| IBIS file stm32mp211_213_215_vfbga361.ibs
[IBIS ver] 5.1
[File name] stm32mp211_213_215_vfbga361.ibs
[File Rev] 0.4
[Date] 09-10-2025
[Source] Data Created at STMicroelectronics
[Notes]  File originated from ELDO simulations.
[Disclaimer]  This information is for modeling purpose only and is
   not guaranted. The information is subject to change without
   notice.
[Copyright] Copyright 2025 STMicroelectronics Inc.
|   Component stm32mp211_213_215_vfbga361
[Component] stm32mp211_213_215_vfbga361
[Manufacturer] STMicroelectronics
[Package]
| variable   typ   min   max
R_pkg  0  NA  NA
L_pkg  0  NA  NA
C_pkg  0  NA  NA
[Pin]   signal_name   model_name
R5  ANA0  nc
P5  ANA1  nc
T2  BOOT0  isudq_tt
P3  BOOT1  isudq_tt
T3  BOOT2  isudq_tt
R3  BOOT3  isudq_tt
C2  CSI_CKN  DPHY_IBIS_L1
C1  CSI_CKP  DPHY_IBIS_L1
E1  CSI_D0N  DPHY_IBIS_L1
E2  CSI_D0P  DPHY_IBIS_L1
D2  CSI_D1N  DPHY_IBIS_L1
D1  CSI_D1P  DPHY_IBIS_L1
E3  CSI_REXT  nc
F17  DDR_A0  mal4drv20_PAD
G17  DDR_A1  mal4drv20_PAD
G18  DDR_A10  mal4drv20_PAD
F18  DDR_A11  mal4drv20_PAD
R17  DDR_A12  mal4drv20_PAD
J18  DDR_A13  mal4drv20_PAD
K18  DDR_A14  mal4drv20_PAD
L18  DDR_A15  mal4drv20_PAD
M18  DDR_A16  mal4drv20_PAD
N18  DDR_A17  mal4drv20_PAD
P18  DDR_A18  mal4drv20_PAD
J17  DDR_A2  mal4drv20_PAD
E19  DDR_A20  mal4drv20_PAD
F19  DDR_A21  mal4drv20_PAD
G19  DDR_A22  mal4drv20_PAD
H19  DDR_A23  mal4drv20_PAD
H17  DDR_A25  mal4drv20_PAD
K19  DDR_A26  mal4drv20_PAD
L19  DDR_A27  mal4drv20_PAD
M19  DDR_A28  mal4drv20_PAD
N19  DDR_A29  mal4drv20_PAD
J19  DDR_A3  mal4drv20_PAD
P19  DDR_A30  mal4drv20_PAD
R19  DDR_A31  mal4drv20_PAD
M17  DDR_A4  mal4drv20_PAD
L17  DDR_A5  mal4drv20_PAD
N17  DDR_A6  mal4drv20_PAD
P17  DDR_A7  mal4drv20_PAD
H18  DDR_A8  mal4drv20_PAD
E18  DDR_A9  mal4drv20_PAD
W18  DDR_DQ0  mal4drv27_PAD
W17  DDR_DQ1  mal4drv27_PAD
B17  DDR_DQ10  mal4drv27_PAD
A17  DDR_DQ11  mal4drv27_PAD
D19  DDR_DQ12  mal4drv27_PAD
D18  DDR_DQ13  mal4drv27_PAD
D17  DDR_DQ14  mal4drv27_PAD
C18  DDR_DQ15  mal4drv27_PAD
V17  DDR_DQ2  mal4drv27_PAD
U17  DDR_DQ3  mal4drv27_PAD
T19  DDR_DQ4  mal4drv27_PAD
T18  DDR_DQ5  mal4drv27_PAD
U19  DDR_DQ6  mal4drv27_PAD
U18  DDR_DQ7  mal4drv27_PAD
C17  DDR_DQ8  mal4drv27_PAD
A18  DDR_DQ9  mal4drv27_PAD
T17  DDR_DQM0  mal4drv27_PAD
C19  DDR_DQM1  mal4drv27_PAD
V18  DDR_DQS0N  mal4drv27_PAD
V19  DDR_DQS0P  mal4drv27_PAD
B18  DDR_DQS1N  mal4drv27_PAD
B19  DDR_DQS1P  mal4drv27_PAD
E17  DDR_RESETN  nc
K17  DDR_VREF  nc
G16  DDR_ZQ  nc
W4  JTCK_SWCLK  io8_tt
W3  JTDI  io8_tt
V1  JTDO_TRACESWO  io8_tt
W2  JTMS_SWDIO  io8_tt
V2  NJTRST  io8_tt
N2  NRST  nc
T1  NRSTC1MS  io8_tt
R1  OSC_IN  isudq_v18
R2  OSC_OUT  isudq_v18
M2  OSC32_IN  isudq_v18
M1  OSC32_OUT  isudq_v18
V12  OTG_HSDM  USB2_HS_IBIS
W12  OTG_HSDP  USB2_HS_IBIS
R15  OTG_TXRTUNE  nc
P15  PA0  io8_tt
N15  PA1  io8_tt_i3c
M15  PA10  io8_tt
R9  PA11  io8_tt
R8  PA12  io8_tt_i3c
W9  PA13  io8_tt
T8  PA14  io8_tt
T10  PA15  io8_tt_i3c
N12  PA2  io8_tt_i3c
R12  PA3  io8_tt_i3c
P12  PA4  io8_tt
J12  PA5  io8_tt
M14  PA6  io8_tt
K15  PA7  io8_tt
K9  PA8  io8_tt_i3c
K12  PA9  io8_tt
D9  PB1  io8_tt
E12  PB10  io8_tt
B7  PB11  io8_tt
E14  PB12  io8_tt
G15  PB13  io8_tt
H15  PB14  io8_tt
J15  PB15  io8_tt
E9  PB2  io8_tt
A9  PB3  io8_tt
B9  PB5  io8_tt_i3c
C8  PB6  io8_tt
D7  PB7  io8_tt
A8  PB9  io8_tt
V9  PC0  io8_tt
V10  PC1  io8_tt_i3c
W6  PC10  io8_tt
V5  PC11  io8_tt
V4  PC12  io8_tt_i3c
P4  PC13  io8_tt
T9  PC2  io8_tt
U4  PC3  io8_tt
V3  PC4  io8_tt
T7  PC5  io8_tt_i3c
R7  PC6  io8_tt_i3c
W5  PC7  io8_tt
U6  PC8  io8_tt
V6  PC9  io8_tt
C11  PD0  io8_tt
F9  PD1  io8_tt
D11  PD10  io8_tt_i3c
B10  PD11  io8_tt_i3c
H14  PD12  io8_tt
G9  PD13  io8_tt
A13  PD14  io8_tt
A11  PD15  io8_tt_i3c
A10  PD2  io8_tt
D8  PD3  io8_tt
C12  PD4  io8_tt
B12  PD5  io8_tt
A12  PD6  io8_tt
D12  PD7  io8_tt
E11  PD8  io8_tt
C10  PD9  io8_tt
N1  PDR_ON  nc
B13  PE0  io8_tt
C13  PE1  io8_tt
D15  PE10  io8_tt
B16  PE11  io8_tt
C16  PE12  io8_tt
A16  PE13  io8_tt
G14  PE14  io8_tt
D14  PE15  io8_tt
A14  PE2  io8_tt
A15  PE3  io8_tt
B14  PE4  io8_tt
C14  PE5  io8_tt
F14  PE6  io8_tt
C15  PE7  io8_tt
B15  PE8  io8_tt
F15  PE9  io8_tt
N9  PF0  io8_tt_i3c
U8  PF1  io8_tt
L9  PF10  io8_tt
T4  PF11  io8_tt
L7  PF12  io8_tt
H2  PF13  io8_tt
G5  PF15  io8_tt
P9  PF2  io8_tt_i3c
W10  PF3  io8_tt
W7  PF4  io8_tt
P7  PF5  io8_tt
U5  PF6  io8_tt
V7  PF7  io8_tt
U7  PF8  io8_tt
T6  PF9  io8_tt
T5  PG0  io8_tt_i3c
R4  PG1  io8_tt_i3c
F5  PG10  io8_tt
F7  PG11  io8_tt
H7  PG12  io8_tt
J7  PG13  io8_tt_i3c
H5  PG14  io8_tt
E4  PG15  io8_tt
M7  PG2  io8_tt_i3c
H12  PG3  io8_tt
N7  PG4  io8_tt
K1  PG5  io8_tt
E7  PG7  io8_tt
E5  PG8  io8_tt
G2  PG9  io8_tt
U10  PH10  io8_tt
T11  PH11  io8_tt
V8  PH12  io8_tt
U9  PH13  io8_tt
G12  PH4  io8_tt
M9  PH5  io8_tt
L12  PH7  io8_tt
M12  PH8  io8_tt
W8  PH9  io8_tt
H1  PI0  io8_tt
J9  PI1  io8_tt_i3c
G1  PI4  io8_tt
K7  PI5  io8_tt
D4  PI6  io8_tt
N4  PI8  io8_tt
P2  PWR_CPUON  io8_tt
P1  PWR_LP  io8_tt
U3  PWR_ON  io8_tt
L5  PZ0  io8_tt_i3c_tamp
M4  PZ1  io8_tt_i3c_tamp
M5  PZ3  io8_tt_i3c_tamp
V11  USBH_HS_DM  USB2_HS_IBIS
W11  USBH_HS_DP  USB2_HS_IBIS
T15  USBH_HS_TXRTUNE  nc
M8  V08CAP  nc
R6  VBAT  power
H8  VDD  power
K8  VDD  power
L6  VDD  power
R14  VDD33USB  power
N6  VDDA18ADC  power
N5  VDDA18AON  power
D3  VDDA18CSI  power
D16  VDDA18DDR  nc
E15  VDDA18PLL1  nc
G6  VDDA18PLL2  nc
T13  VDDA18USB  power
G10  VDDCORE  nc
H11  VDDCORE  nc
J10  VDDCORE  nc
K11  VDDCORE  nc
L10  VDDCORE  nc
M11  VDDCORE  nc
N8  VDDCORE  nc
N10  VDDCORE  nc
N14  VDDCORE  nc
P11  VDDCORE  nc
P13  VDDCORE  nc
R10  VDDCORE  nc
E13  VDDCPU  nc
G13  VDDCPU  nc
J13  VDDCPU  nc
L13  VDDCPU  nc
M13  VDDCPU  nc
B1  VDDCSI  nc
D10  VDDIO1  power
F8  VDDIO2  power
E10  VDDIO3  power
F10  VDDIO3  power
F16  VDDQDDR  power
J16  VDDQDDR  power
L16  VDDQDDR  power
M16  VDDQDDR  power
P16  VDDQDDR  power
T16  VDDQDDR  power
U1  VREFN  nc
U2  VREFP  nc
A1  VSS  gnd
A19  VSS  gnd
C3  VSS  gnd
C7  VSS  gnd
D13  VSS  gnd
E8  VSS  gnd
E16  VSS  gnd
F6  VSS  gnd
F11  VSS  gnd
F13  VSS  gnd
G8  VSS  gnd
G11  VSS  gnd
H10  VSS  gnd
H13  VSS  gnd
H16  VSS  gnd
J6  VSS  gnd
J8  VSS  gnd
J11  VSS  gnd
J14  VSS  gnd
K4  VSS  gnd
K5  VSS  gnd
K10  VSS  gnd
K13  VSS  gnd
K16  VSS  gnd
L8  VSS  gnd
L11  VSS  gnd
M10  VSS  gnd
N11  VSS  gnd
N13  VSS  gnd
N16  VSS  gnd
P8  VSS  gnd
P10  VSS  gnd
P14  VSS  gnd
R11  VSS  gnd
R16  VSS  gnd
R18  VSS  gnd
W1  VSS  gnd
W19  VSS  gnd
P6  VSSA  nc
M6  VSSAON  nc
[Package Model]   503-fcvfbga-10x10-361-240814
[Pin Mapping]   pulldown_ref   pullup_ref   | Comment
R5  nc  nc
P5  nc  nc
T2  gnd  vdd
P3  gnd  vdd
T3  gnd  vdd
R3  gnd  vdd
C2  gnd  VDDA18CSI
C1  gnd  VDDA18CSI
E1  gnd  VDDA18CSI
E2  gnd  VDDA18CSI
D2  gnd  VDDA18CSI
D1  gnd  VDDA18CSI
E3  nc  nc
F17  gnd  vddqddr
G17  gnd  vddqddr
G18  gnd  vddqddr
F18  gnd  vddqddr
R17  gnd  vddqddr
J18  gnd  vddqddr
K18  gnd  vddqddr
L18  gnd  vddqddr
M18  gnd  vddqddr
N18  gnd  vddqddr
P18  gnd  vddqddr
J17  gnd  vddqddr
E19  gnd  vddqddr
F19  gnd  vddqddr
G19  gnd  vddqddr
H19  gnd  vddqddr
H17  gnd  vddqddr
K19  gnd  vddqddr
L19  gnd  vddqddr
M19  gnd  vddqddr
N19  gnd  vddqddr
J19  gnd  vddqddr
P19  gnd  vddqddr
R19  gnd  vddqddr
M17  gnd  vddqddr
L17  gnd  vddqddr
N17  gnd  vddqddr
P17  gnd  vddqddr
H18  gnd  vddqddr
E18  gnd  vddqddr
W18  gnd  vddqddr
W17  gnd  vddqddr
B17  gnd  vddqddr
A17  gnd  vddqddr
D19  gnd  vddqddr
D18  gnd  vddqddr
D17  gnd  vddqddr
C18  gnd  vddqddr
V17  gnd  vddqddr
U17  gnd  vddqddr
T19  gnd  vddqddr
T18  gnd  vddqddr
U19  gnd  vddqddr
U18  gnd  vddqddr
C17  gnd  vddqddr
A18  gnd  vddqddr
T17  gnd  vddqddr
C19  gnd  vddqddr
V18  gnd  vddqddr
V19  gnd  vddqddr
B18  gnd  vddqddr
B19  gnd  vddqddr
E17  nc  nc
K17  nc  nc
G16  nc  nc
W4  gnd  vdd
W3  gnd  vdd
V1  gnd  vdd
W2  gnd  vdd
V2  gnd  vdd
N2  nc  nc
T1  gnd  vdd
R1  gnd  vdda18aon
R2  gnd  vdda18aon
M2  gnd  vdd  | Depending on IO usage
| M2  gnd  vsw  | Depending on IO usage
M1  gnd  vdd  | Depending on IO usage
| M1  gnd  vsw  | Depending on IO usage
V12  gnd  VDD33USB
W12  gnd  VDD33USB
R15  nc  nc
P15  gnd  vdd
N15  gnd  vdd
M15  gnd  vdd
R9  gnd  vdd
R8  gnd  vdd
W9  gnd  vdd
T8  gnd  vdd
T10  gnd  vdd
N12  gnd  vdd
R12  gnd  vdd
P12  gnd  vdd
J12  gnd  vdd
M14  gnd  vdd
K15  gnd  vdd
K9  gnd  vdd
K12  gnd  vdd
D9  gnd  vdd
E12  gnd  vdd
B7  gnd  vdd
E14  gnd  vdd
G15  gnd  vdd
H15  gnd  vdd
J15  gnd  vdd
E9  gnd  vdd
A9  gnd  vdd
B9  gnd  vdd
C8  gnd  vdd
D7  gnd  vdd
A8  gnd  vdd
V9  gnd  vdd
V10  gnd  vdd
W6  gnd  vdd
V5  gnd  vdd
V4  gnd  vdd
P4  gnd  vdd  | Depending on IO usage
| P4  gnd  vsw  | Depending on IO usage
T9  gnd  vdd
U4  gnd  vdd
V3  gnd  vdd
T7  gnd  vdd
R7  gnd  vdd
W5  gnd  vdd
U6  gnd  vdd
V6  gnd  vdd
C11  gnd  vddio3
F9  gnd  vddio3
D11  gnd  vddio3
B10  gnd  vddio3
H14  gnd  vdd
G9  gnd  vdd
A13  gnd  vdd
A11  gnd  vdd
A10  gnd  vddio3
D8  gnd  vddio3
C12  gnd  vddio3
B12  gnd  vddio3
A12  gnd  vddio3
D12  gnd  vddio3
E11  gnd  vddio3
C10  gnd  vddio3
N1  nc  nc
B13  gnd  vddio1
C13  gnd  vddio1
D15  gnd  vddio2
B16  gnd  vddio2
C16  gnd  vddio2
A16  gnd  vddio2
G14  gnd  vddio2
D14  gnd  vddio2
A14  gnd  vddio1
A15  gnd  vddio1
B14  gnd  vddio1
C14  gnd  vddio1
F14  gnd  vddio1
C15  gnd  vddio1
B15  gnd  vddio1
F15  gnd  vddio1
N9  gnd  vdd
U8  gnd  vdd
L9  gnd  vdd
T4  gnd  vdd
L7  gnd  vdd
H2  gnd  vdd
G5  gnd  vdd
P9  gnd  vdd
W10  gnd  vdd
W7  gnd  vdd
P7  gnd  vdd
U5  gnd  vdd
V7  gnd  vdd
U7  gnd  vdd
T6  gnd  vdd
T5  gnd  vdd
R4  gnd  vdd
F5  gnd  vdd
F7  gnd  vdd
H7  gnd  vdd
J7  gnd  vdd
H5  gnd  vdd
E4  gnd  vdd
M7  gnd  vdd
H12  gnd  vdd
N7  gnd  vdd
K1  gnd  vdd
E7  gnd  vdd
E5  gnd  vdd
G2  gnd  vdd
U10  gnd  vdd
T11  gnd  vdd
V8  gnd  vdd
U9  gnd  vdd
G12  gnd  vdd
M9  gnd  vdd
L12  gnd  vdd
M12  gnd  vdd
W8  gnd  vdd
H1  gnd  vdd
J9  gnd  vdd
G1  gnd  vdd
K7  gnd  vdd
D4  gnd  vdd
N4  gnd  vdd
P2  gnd  vdd
P1  gnd  vdd
U3  gnd  vdd
L5  gnd  vdd  | Depending on IO usage
| L5  gnd  vsw  | Depending on IO usage
M4  gnd  vdd  | Depending on IO usage
| M4  gnd  vsw  | Depending on IO usage
M5  gnd  vdd  | Depending on IO usage
| M5  gnd  vsw  | Depending on IO usage
V11  gnd  VDD33USB
W11  gnd  VDD33USB
T15  nc  nc
M8  nc  nc
R6  nc  vsw
H8  nc  vdd
K8  nc  vdd
L6  nc  vdd
R14  nc  VDD33USB
N6  nc  vdda18adc
N5  nc  vdda18aon
D3  nc  VDDA18CSI
D16  nc  nc
E15  nc  nc
G6  nc  nc
T13  nc  vdda18usb
G10  nc  nc
H11  nc  nc
J10  nc  nc
K11  nc  nc
L10  nc  nc
M11  nc  nc
N8  nc  nc
N10  nc  nc
N14  nc  nc
P11  nc  nc
P13  nc  nc
R10  nc  nc
E13  nc  nc
G13  nc  nc
J13  nc  nc
L13  nc  nc
M13  nc  nc
B1  nc  nc
D10  nc  vddio1
F8  nc  vddio2
E10  nc  vddio3
F10  nc  vddio3
F16  nc  vddqddr
J16  nc  vddqddr
L16  nc  vddqddr
M16  nc  vddqddr
P16  nc  vddqddr
T16  nc  vddqddr
U1  nc  nc
U2  nc  nc
A1  gnd  nc
A19  gnd  nc
C3  gnd  nc
C7  gnd  nc
D13  gnd  nc
E8  gnd  nc
E16  gnd  nc
F6  gnd  nc
F11  gnd  nc
F13  gnd  nc
G8  gnd  nc
G11  gnd  nc
H10  gnd  nc
H13  gnd  nc
H16  gnd  nc
J6  gnd  nc
J8  gnd  nc
J11  gnd  nc
J14  gnd  nc
K4  gnd  nc
K5  gnd  nc
K10  gnd  nc
K13  gnd  nc
K16  gnd  nc
L8  gnd  nc
L11  gnd  nc
M10  gnd  nc
N11  gnd  nc
N13  gnd  nc
N16  gnd  nc
P8  gnd  nc
P10  gnd  nc
P14  gnd  nc
R11  gnd  nc
R16  gnd  nc
R18  gnd  nc
W1  gnd  nc
W19  gnd  nc
P6  nc  nc
M6  nc  nc
[Diff Pin]  inv_pin  vdiff  tdelay_typ  tdelay_min  tdelay_max
C2  C1  NA  NA  NA  NA
E1  E2  NA  NA  NA  NA
D2  D1  NA  NA  NA  NA
V19  V18  NA  NA  NA  NA
B19  B18  NA  NA  NA  NA
W11  V11  NA  NA  NA  NA   |USBH_HS_DP _DM
W12  V12  NA  NA  NA  NA   |USBH_HS_DP _DM
M17  L17  NA  NA  NA  NA
[Model Selector] USB2_HS_IBIS
USB2_HSRX   USB2 HSRX model
USB2_HSTX_00_0_01_0011_11   TuningBits_AMP_PULSE_RISE_REF_XV=00_0_01_0011_11
USB2_HSTX_00_0_10_0101_11   TuningBits_AMP_PULSE_RISE_REF_XV=00_0_10_0101_11
USB2_HSTX_00_0_11_0111_11   TuningBits_AMP_PULSE_RISE_REF_XV=00_0_11_0111_11
USB2_HSTX_00_1_01_0011_11   TuningBits_AMP_PULSE_RISE_REF_XV=00_1_01_0011_11
USB2_HSTX_00_1_10_0101_11   TuningBits_AMP_PULSE_RISE_REF_XV=00_1_10_0101_11
USB2_HSTX_00_1_11_0111_11   TuningBits_AMP_PULSE_RISE_REF_XV=00_1_11_0111_11
USB2_HSTX_01_0_01_0011_11   TuningBits_AMP_PULSE_RISE_REF_XV=01_0_01_0011_11
USB2_HSTX_01_0_10_0101_11   TuningBits_AMP_PULSE_RISE_REF_XV=01_0_10_0101_11
USB2_HSTX_01_0_11_0111_11   TuningBits_AMP_PULSE_RISE_REF_XV=01_0_11_0111_11
USB2_HSTX_01_1_01_0011_11   TuningBits_AMP_PULSE_RISE_REF_XV=01_1_01_0011_11
USB2_HSTX_01_1_10_0101_11   TuningBits_AMP_PULSE_RISE_REF_XV=01_1_10_0101_11
USB2_HSTX_01_1_11_0111_11   TuningBits_AMP_PULSE_RISE_REF_XV=01_1_11_0111_11
USB2_HSTX_10_0_01_0011_11   TuningBits_AMP_PULSE_RISE_REF_XV=10_0_01_0011_11
USB2_HSTX_10_0_10_0101_11   TuningBits_AMP_PULSE_RISE_REF_XV=10_0_10_0101_11
USB2_HSTX_10_0_11_0111_11   TuningBits_AMP_PULSE_RISE_REF_XV=10_0_11_0111_11
USB2_HSTX_10_1_01_0011_11   TuningBits_AMP_PULSE_RISE_REF_XV=10_1_01_0011_11
USB2_HSTX_10_1_10_0101_11   TuningBits_AMP_PULSE_RISE_REF_XV=10_1_10_0101_11
USB2_HSTX_10_1_11_0111_11   TuningBits_AMP_PULSE_RISE_REF_XV=10_1_11_0111_11
[Model Selector] DPHY_IBIS_L1
DPHY_RX_2P5G_L1   DPHY HSRX model at 2.5Gbps for lane 1
DPHY_RX_1P5G_L1   DPHY HSRX model at 1.5Gbps for lane 1
[Model Selector] io8_tt
io8_tt_ls_3v3 "GPIO - 3V tolerant - low speed - 3.3V range"
io8_tt_ms_3v3 "GPIO - 3V tolerant - med speed - 3.3V range"
io8_tt_fs_3v3 "GPIO - 3V tolerant - fast speed - 3.3V range"
io8_tt_hs_3v3 "GPIO - 3V tolerant - high speed - 3.3V range"
io8_tt_hslv_ls_1v8 "GPIO low voltage optimization - 3V tolerant - low speed - 1.8V range"
io8_tt_hslv_ms_1v8 "GPIO low voltage optimization - 3V tolerant - med speed - 1.8V range"
io8_tt_hslv_fs_1v8 "GPIO low voltage optimization - 3V tolerant - fast speed - 1.8V range"
io8_tt_hslv_hs_1v8 "GPIO low voltage optimization - 3V tolerant - high speed - 1.8V range"
[Model Selector] io8_tt_i3c
io8_tt_ls_3v3 "GPIO - 3V tolerant - low speed - 3.3V range"
io8_tt_ms_3v3 "GPIO - 3V tolerant - med speed - 3.3V range"
io8_tt_fs_3v3 "GPIO - 3V tolerant - fast speed - 3.3V range"
io8_tt_hs_3v3 "GPIO - 3V tolerant - high speed - 3.3V range"
io8_tt_hslv_ls_1v8 "GPIO low voltage optimization - 3V tolerant - low speed - 1.8V range"
io8_tt_hslv_ms_1v8 "GPIO low voltage optimization - 3V tolerant - med speed - 1.8V range"
io8_tt_hslv_fs_1v8 "GPIO low voltage optimization - 3V tolerant - fast speed - 1.8V range"
io8_tt_hslv_hs_1v8 "GPIO low voltage optimization - 3V tolerant - high speed - 1.8V range"
io8_tt_i3c_ls_3v3 "GPIO with I3C open-drain - 3V tolerant - low speed - 3.3V range"
io8_tt_i3c_ms_3v3 "GPIO with I3C open-drain - 3V tolerant - med speed - 3.3V range"
io8_tt_i3c_fs_3v3 "GPIO with I3C open-drain - 3V tolerant - fast speed - 3.3V range"
io8_tt_i3c_hs_3v3 "GPIO with I3C open-drain - 3V tolerant - high speed - 3.3V range"
io8_tt_hslv_i3c_ls_1v8 "GPIO low voltage optimization with I3C open-drain - 3V tolerant - low speed - 1.8V range"
io8_tt_hslv_i3c_ms_1v8 "GPIO low voltage optimization with I3C open-drain - 3V tolerant - med speed - 1.8V range"
io8_tt_hslv_i3c_fs_1v8 "GPIO low voltage optimization with I3C open-drain - 3V tolerant - fast speed - 1.8V range"
io8_tt_hslv_i3c_hs_1v8 "GPIO low voltage optimization with I3C open-drain - 3V tolerant - high speed - 1.8V range"
io8_tt_i3c_fmp_3v3 "GPIO with I3C fm+ open-drain - 3V tolerant - 3.3V range"
[Model Selector] io8_tt_i3c_tamp
io8_tt_ls_3v3 "GPIO - 3V tolerant - low speed - 3.3V range"
io8_tt_ms_3v3 "GPIO - 3V tolerant - med speed - 3.3V range"
io8_tt_fs_3v3 "GPIO - 3V tolerant - fast speed - 3.3V range"
io8_tt_hs_3v3 "GPIO - 3V tolerant - high speed - 3.3V range"
io8_tt_hslv_ls_1v8 "GPIO low voltage optimization - 3V tolerant - low speed - 1.8V range"
io8_tt_hslv_ms_1v8 "GPIO low voltage optimization - 3V tolerant - med speed - 1.8V range"
io8_tt_hslv_fs_1v8 "GPIO low voltage optimization - 3V tolerant - fast speed - 1.8V range"
io8_tt_hslv_hs_1v8 "GPIO low voltage optimization - 3V tolerant - high speed - 1.8V range"
io8_tt_i3c_ls_3v3 "GPIO with I3C open-drain - 3V tolerant - low speed - 3.3V range"
io8_tt_i3c_ms_3v3 "GPIO with I3C open-drain - 3V tolerant - med speed - 3.3V range"
io8_tt_i3c_fs_3v3 "GPIO with I3C open-drain - 3V tolerant - fast speed - 3.3V range"
io8_tt_i3c_hs_3v3 "GPIO with I3C open-drain - 3V tolerant - high speed - 3.3V range"
io8_tt_hslv_i3c_ls_1v8 "GPIO low voltage optimization with I3C open-drain - 3V tolerant - low speed - 1.8V range"
io8_tt_hslv_i3c_ms_1v8 "GPIO low voltage optimization with I3C open-drain - 3V tolerant - med speed - 1.8V range"
io8_tt_hslv_i3c_fs_1v8 "GPIO low voltage optimization with I3C open-drain - 3V tolerant - fast speed - 1.8V range"
io8_tt_hslv_i3c_hs_1v8 "GPIO low voltage optimization with I3C open-drain - 3V tolerant - high speed - 1.8V range"
io8_tt_i3c_fmp_3v3 "GPIO with I3C fm+ open-drain - 3V tolerant - 3.3V range"
io8_tt_tamp_3v3 "IO tamper - 3V tolerant - 3.3V range"
io8_tt_tamp_1v8 "IO tamper - 3V tolerant - 1.8V range"
[Model Selector] isudq_tt
isudq_tt_3v3 "Input Buffer - 3V tolerant - 3.3V range"
isudq_tt_1v8 "Input Buffer - 3V tolerant - 1.8V range"
|[Model Selector] isudq_v18
|isudq_v18_1v8 "Input Buffer - 1.8V range "
[Model Selector]   mal4drv20_PAD
mal4drv20_d3l_40   DDR3L mal4drv20 cell  Z0=40-Ohm Driver
mal4drv20_d3l_60   DDR3L mal4drv20 cell  Z0=60-Ohm Driver
mal4drv20_d3l_120   DDR3L mal4drv20 cell  Z0=120-Ohm Driver
mal4drv20_d3_20   DDR3 mal4drv20 cell  Z0=20-Ohm Driver
mal4drv20_d3_24   DDR3 mal4drv20 cell  Z0=24-Ohm Driver
mal4drv20_d3_30   DDR3 mal4drv20 cell  Z0=30-Ohm Driver
mal4drv20_d3_40   DDR3 mal4drv20 cell  Z0=40-Ohm Driver
mal4drv20_d3_60   DDR3 mal4drv20 cell  Z0=60-Ohm Driver
mal4drv20_d4_20   DDR4 mal4drv20 cell  Z0=20-Ohm Driver
mal4drv20_d4_24   DDR4 mal4drv20 cell  Z0=24-Ohm Driver
mal4drv20_d4_30   DDR4 mal4drv20 cell  Z0=30-Ohm Driver
mal4drv20_d4_40   DDR4 mal4drv20 cell  Z0=40-Ohm Driver
mal4drv20_d4_60   DDR4 mal4drv20 cell  Z0=60-Ohm Driver
mal4drv20_dl4_20   LPDDR4 mal4drv20 cell  Z0=20-Ohm Driver
mal4drv20_dl4_24   LPDDR4 mal4drv20 cell  Z0=24-Ohm Driver
mal4drv20_dl4_30   LPDDR4 mal4drv20 cell  Z0=30-Ohm Driver
mal4drv20_dl4_40   LPDDR4 mal4drv20 cell  Z0=40-Ohm Driver
mal4drv20_dl4_60   LPDDR4 mal4drv20 cell  Z0=60-Ohm Driver
[Model Selector]   mal4drv27_PAD
mal4drv27_d3l_40   DDR3L mal4drv27 cell  Z0=40-Ohm Driver
mal4drv27_d3l_48   DDR3L mal4drv27 cell  Z0=48-Ohm Driver
mal4drv27_d3l_60   DDR3L mal4drv27 cell  Z0=60-Ohm Driver
mal4drv27_d3l_80   DDR3L mal4drv27 cell  Z0=80-Ohm Driver
mal4drv27_d3l_120   DDR3L mal4drv27 cell  Z0=120-Ohm Driver
mal4drv27_d3l_240   DDR3L mal4drv27 cell  Z0=240-Ohm Driver
mal4drv27_d3l_odt120   DDR3L mal4drv27 cell 120-Ohm ODT Receiver
mal4drv27_d3l_odt60   DDR3L mal4drv27 cell 60-Ohm ODT Receiver
mal4drv27_d3l_odtoff   DDR3L mal4drv27 cell ODT OFF Receiver
mal4drv27_d3_28   DDR3 mal4drv27 cell  Z0=28-Ohm Driver
mal4drv27_d3_34   DDR3 mal4drv27 cell  Z0=34-Ohm Driver
mal4drv27_d3_40   DDR3 mal4drv27 cell  Z0=40-Ohm Driver
mal4drv27_d3_53   DDR3 mal4drv27 cell  Z0=53-Ohm Driver
mal4drv27_d3_odt120   DDR3 mal4drv27 cell 120-Ohm ODT Receiver
mal4drv27_d3_odt60   DDR3 mal4drv27 cell 60-Ohm ODT Receiver
mal4drv27_d4_28   DDR4 mal4drv27 cell  Z0=28-Ohm Driver
mal4drv27_d4_34   DDR4 mal4drv27 cell  Z0=34-Ohm Driver
mal4drv27_d4_40   DDR4 mal4drv27 cell  Z0=40-Ohm Driver
mal4drv27_d4_53   DDR4 mal4drv27 cell  Z0=53-Ohm Driver
mal4drv27_d4_odt120   DDR4 mal4drv27 cell 120-Ohm ODT Receiver
mal4drv27_d4_odt240   DDR4 mal4drv27 cell 240-Ohm ODT Receiver
mal4drv27_d4_odt48   DDR4 mal4drv27 cell 48-Ohm ODT Receiver
mal4drv27_d4_odt60   DDR4 mal4drv27 cell 60-Ohm ODT Receiver
mal4drv27_d4_odt80   DDR4 mal4drv27 cell 80-Ohm ODT Receiver
mal4drv27_dl4_28   LPDDR4 mal4drv27 cell  Z0=28-Ohm Driver
mal4drv27_dl4_34   LPDDR4 mal4drv27 cell  Z0=34-Ohm Driver
mal4drv27_dl4_40   LPDDR4 mal4drv27 cell  Z0=40-Ohm Driver
mal4drv27_dl4_53   LPDDR4 mal4drv27 cell  Z0=53-Ohm Driver
mal4drv27_dl4_odt48   LPDDR4 mal4drv27 cell 48-Ohm ODT Receiver
mal4drv27_dl4_odt60   LPDDR4 mal4drv27 cell 60-Ohm ODT Receiver
[Define Package Model]  503-fcvfbga-10x10-361-240814
[Manufacturer]  unknown
[OEM]  unknown
[Description]  unknown
[Number Of Pins]  235
[Pin Numbers]
| Pin Name Terminal   Net Name   Starting Node   Ending Node
R5 | ANA0
P5 | ANA1
T2 | BOOT0
P3 | BOOT1
T3 | BOOT2
R3 | BOOT3
C2 | CSI_CKN
C1 | CSI_CKP
E1 | CSI_D0N
E2 | CSI_D0P
D2 | CSI_D1N
D1 | CSI_D1P
E3 | CSI_REXT
F17 | DDR_A0
G17 | DDR_A1
J17 | DDR_A2
J19 | DDR_A3
M17 | DDR_A4
L17 | DDR_A5
N17 | DDR_A6
P17 | DDR_A7
H18 | DDR_A8
E18 | DDR_A9
G18 | DDR_A10
F18 | DDR_A11
R17 | DDR_A12
J18 | DDR_A13
K18 | DDR_A14
L18 | DDR_A15
M18 | DDR_A16
N18 | DDR_A17
P18 | DDR_A18
E19 | DDR_A20
F19 | DDR_A21
G19 | DDR_A22
H19 | DDR_A23
H17 | DDR_A25
K19 | DDR_A26
L19 | DDR_A27
M19 | DDR_A28
N19 | DDR_A29
P19 | DDR_A30
R19 | DDR_A31
W18 | DDR_DQ0
W17 | DDR_DQ1
V17 | DDR_DQ2
U17 | DDR_DQ3
T19 | DDR_DQ4
T18 | DDR_DQ5
U19 | DDR_DQ6
U18 | DDR_DQ7
C17 | DDR_DQ8
A18 | DDR_DQ9
B17 | DDR_DQ10
A17 | DDR_DQ11
D19 | DDR_DQ12
D18 | DDR_DQ13
D17 | DDR_DQ14
C18 | DDR_DQ15
T17 | DDR_DQM0
C19 | DDR_DQM1
V18 | DDR_DQS0N
V19 | DDR_DQS0P
B18 | DDR_DQS1N
B19 | DDR_DQS1P
E17 | DDR_RESETN
K17 | DDR_VREF
G16 | DDR_ZQ
W4 | JTCK_SWCLK
W3 | JTDI
V1 | JTDO_TRACESWO
W2 | JTMS_SWDIO
V2 | NJTRST
N2 | NRST
T1 | NRSTC1MS
M2 | OSC32_IN
M1 | OSC32_OUT
R1 | OSC_IN
R2 | OSC_OUT
V12 | OTG_HSDM
W12 | OTG_HSDP
R15 | OTG_TXRTUNE
P15 | PA0
N15 | PA1
N12 | PA2
R12 | PA3
P12 | PA4
J12 | PA5
M14 | PA6
K15 | PA7
K9 | PA8
K12 | PA9
M15 | PA10
R9 | PA11
R8 | PA12
W9 | PA13
T8 | PA14
T10 | PA15
D9 | PB1
E9 | PB2
A9 | PB3
B9 | PB5
C8 | PB6
D7 | PB7
A8 | PB9
E12 | PB10
B7 | PB11
E14 | PB12
G15 | PB13
H15 | PB14
J15 | PB15
V9 | PC0
V10 | PC1
T9 | PC2
U4 | PC3
V3 | PC4
T7 | PC5
R7 | PC6
W5 | PC7
U6 | PC8
V6 | PC9
W6 | PC10
V5 | PC11
V4 | PC12
P4 | PC13
C11 | PD0
F9 | PD1
A10 | PD2
D8 | PD3
C12 | PD4
B12 | PD5
A12 | PD6
D12 | PD7
E11 | PD8
C10 | PD9
D11 | PD10
B10 | PD11
H14 | PD12
G9 | PD13
A13 | PD14
A11 | PD15
N1 | PDR_ON
B13 | PE0
C13 | PE1
A14 | PE2
A15 | PE3
B14 | PE4
C14 | PE5
F14 | PE6
C15 | PE7
B15 | PE8
F15 | PE9
D15 | PE10
B16 | PE11
C16 | PE12
A16 | PE13
G14 | PE14
D14 | PE15
N9 | PF0
U8 | PF1
P9 | PF2
W10 | PF3
W7 | PF4
P7 | PF5
U5 | PF6
V7 | PF7
U7 | PF8
T6 | PF9
L9 | PF10
T4 | PF11
L7 | PF12
H2 | PF13
G5 | PF15
T5 | PG0
R4 | PG1
M7 | PG2
H12 | PG3
N7 | PG4
K1 | PG5
E7 | PG7
E5 | PG8
G2 | PG9
F5 | PG10
F7 | PG11
H7 | PG12
J7 | PG13
H5 | PG14
E4 | PG15
G12 | PH4
M9 | PH5
L12 | PH7
M12 | PH8
W8 | PH9
U10 | PH10
T11 | PH11
V8 | PH12
U9 | PH13
H1 | PI0
J9 | PI1
G1 | PI4
K7 | PI5
D4 | PI6
N4 | PI8
P2 | PWR_CPUON
P1 | PWR_LP
U3 | PWR_ON
L5 | PZ0
M4 | PZ1
M5 | PZ3
V11 | USBH_HS_DM
W11 | USBH_HS_DP
T15 | USBH_HS_TXRTUNE
M8 | V08CAP
R6 | VBAT
R14 | VDD33USB
H8 | VDD
N6 | VDDA18ADC
N5 | VDDA18AON
D3 | VDDA18CSI
D16 | VDDA18DDR
E15 | VDDA18PLL1
G6 | VDDA18PLL2
T13 | VDDA18USB
G10 | VDDCORE
E13 | VDDCPU
B1 | VDDCSI
D10 | VDDIO1
F8 | VDDIO2
E10 | VDDIO3
F16 | VDDQDDR
U1 | VREFN
U2 | VREFP
A1 | VSS
P6 | VSSA
M6 | VSSAON
|[Merged Pins]  H8
|K8  |  VDD
|L6  |  VDD
|[Merged Pins]  G10
|H11  |  VDDCORE
|J10  |  VDDCORE
|K11  |  VDDCORE
|L10  |  VDDCORE
|M11  |  VDDCORE
|N8  |  VDDCORE
|N10  |  VDDCORE
|N14  |  VDDCORE
|P11  |  VDDCORE
|P13  |  VDDCORE
|R10  |  VDDCORE
|[Merged Pins]  E13
|G13  |  VDDCPU
|J13  |  VDDCPU
|L13  |  VDDCPU
|M13  |  VDDCPU
|[Merged Pins]  E10
|F10  |  VDDIO3
|[Merged Pins]  F16
|J16  |  VDDQDDR
|L16  |  VDDQDDR
|M16  |  VDDQDDR
|P16  |  VDDQDDR
|T16  |  VDDQDDR
|[Merged Pins]  A1
|A19  |  VSS
|C3  |  VSS
|C7  |  VSS
|D13  |  VSS
|E8  |  VSS
|E16  |  VSS
|F6  |  VSS
|F11  |  VSS
|F13  |  VSS
|G8  |  VSS
|G11  |  VSS
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[Model Data]
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[End Model Data]
[End Package Model]
|End [Component]
| Models and submodels in the file (91): USB2_HSRX (Input), USB2_HSTX_00_0_01_0011_11 (Output), USB2_HSTX_00_0_10_0101_11 (Output), USB2_HSTX_00_0_11_0111_11 (Output), USB2_HSTX_00_1_01_0011_11 (Output), USB2_HSTX_00_1_10_0101_11 (Output), USB2_HSTX_00_1_11_0111_11 (Output), USB2_HSTX_01_0_01_0011_11 (Output), USB2_HSTX_01_0_10_0101_11 (Output), USB2_HSTX_01_0_11_0111_11 (Output), USB2_HSTX_01_1_01_0011_11 (Output), USB2_HSTX_01_1_10_0101_11 (Output), USB2_HSTX_01_1_11_0111_11 (Output), USB2_HSTX_10_0_01_0011_11 (Output), USB2_HSTX_10_0_10_0101_11 (Output), USB2_HSTX_10_0_11_0111_11 (Output), USB2_HSTX_10_1_01_0011_11 (Output), USB2_HSTX_10_1_10_0101_11 (Output), USB2_HSTX_10_1_11_0111_11 (Output), DPHY_RX_1P5G_L1 (Input), DPHY_RX_2P5G_L1 (Input), mal4drv20_d3_20 (I/O), mal4drv20_d3_24 (I/O), mal4drv20_d3_30 (I/O), mal4drv20_d3_40 (I/O), mal4drv20_d3_60 (I/O), mal4drv20_d4_20 (I/O), mal4drv20_d4_24 (I/O), mal4drv20_d4_30 (I/O), mal4drv20_d4_40 (I/O), mal4drv20_d4_60 (I/O), mal4drv20_dl4_20 (I/O), mal4drv20_dl4_24 (I/O), mal4drv20_dl4_30 (I/O), mal4drv20_dl4_40 (I/O), mal4drv20_dl4_60 (I/O), mal4drv27_d3_28 (I/O), mal4drv27_d3_34 (I/O), mal4drv27_d3_40 (I/O), mal4drv27_d3_53 (I/O), mal4drv27_d3_odt120 (Input), mal4drv27_d3_odt60 (Input), mal4drv27_dl4_28 (I/O), mal4drv27_dl4_34 (I/O), mal4drv27_dl4_40 (I/O), mal4drv27_dl4_53 (I/O), mal4drv27_dl4_odt48 (Input), mal4drv27_dl4_odt60 (Input), mal4drv27_d4_28 (I/O), mal4drv27_d4_34 (I/O), mal4drv27_d4_40 (I/O), mal4drv27_d4_53 (I/O), mal4drv27_d4_odt120 (Input), mal4drv27_d4_odt240 (Input), mal4drv27_d4_odt48 (Input), mal4drv27_d4_odt60 (Input), mal4drv27_d4_odt80 (Input), mal4drv20_d3l_120 (I/O), mal4drv20_d3l_40 (I/O), mal4drv20_d3l_60 (I/O), mal4drv27_d3l_120 (I/O), mal4drv27_d3l_240 (I/O), mal4drv27_d3l_40 (I/O), mal4drv27_d3l_48 (I/O), mal4drv27_d3l_60 (I/O), mal4drv27_d3l_80 (I/O), mal4drv27_d3l_odt120 (Input), mal4drv27_d3l_odt60 (Input), mal4drv27_d3l_odtoff (Input), io8_tt_fs_3v3 (I/O), io8_tt_hs_3v3 (I/O), io8_tt_hslv_fs_1v8 (I/O), io8_tt_hslv_hs_1v8 (I/O), io8_tt_hslv_i3c_fs_1v8 (I/O_open_drain), io8_tt_hslv_i3c_hs_1v8 (I/O_open_drain), io8_tt_hslv_i3c_ls_1v8 (I/O_open_drain), io8_tt_hslv_i3c_ms_1v8 (I/O_open_drain), io8_tt_hslv_ls_1v8 (I/O), io8_tt_hslv_ms_1v8 (I/O), io8_tt_i3c_fmp_3v3 (I/O_open_drain)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
